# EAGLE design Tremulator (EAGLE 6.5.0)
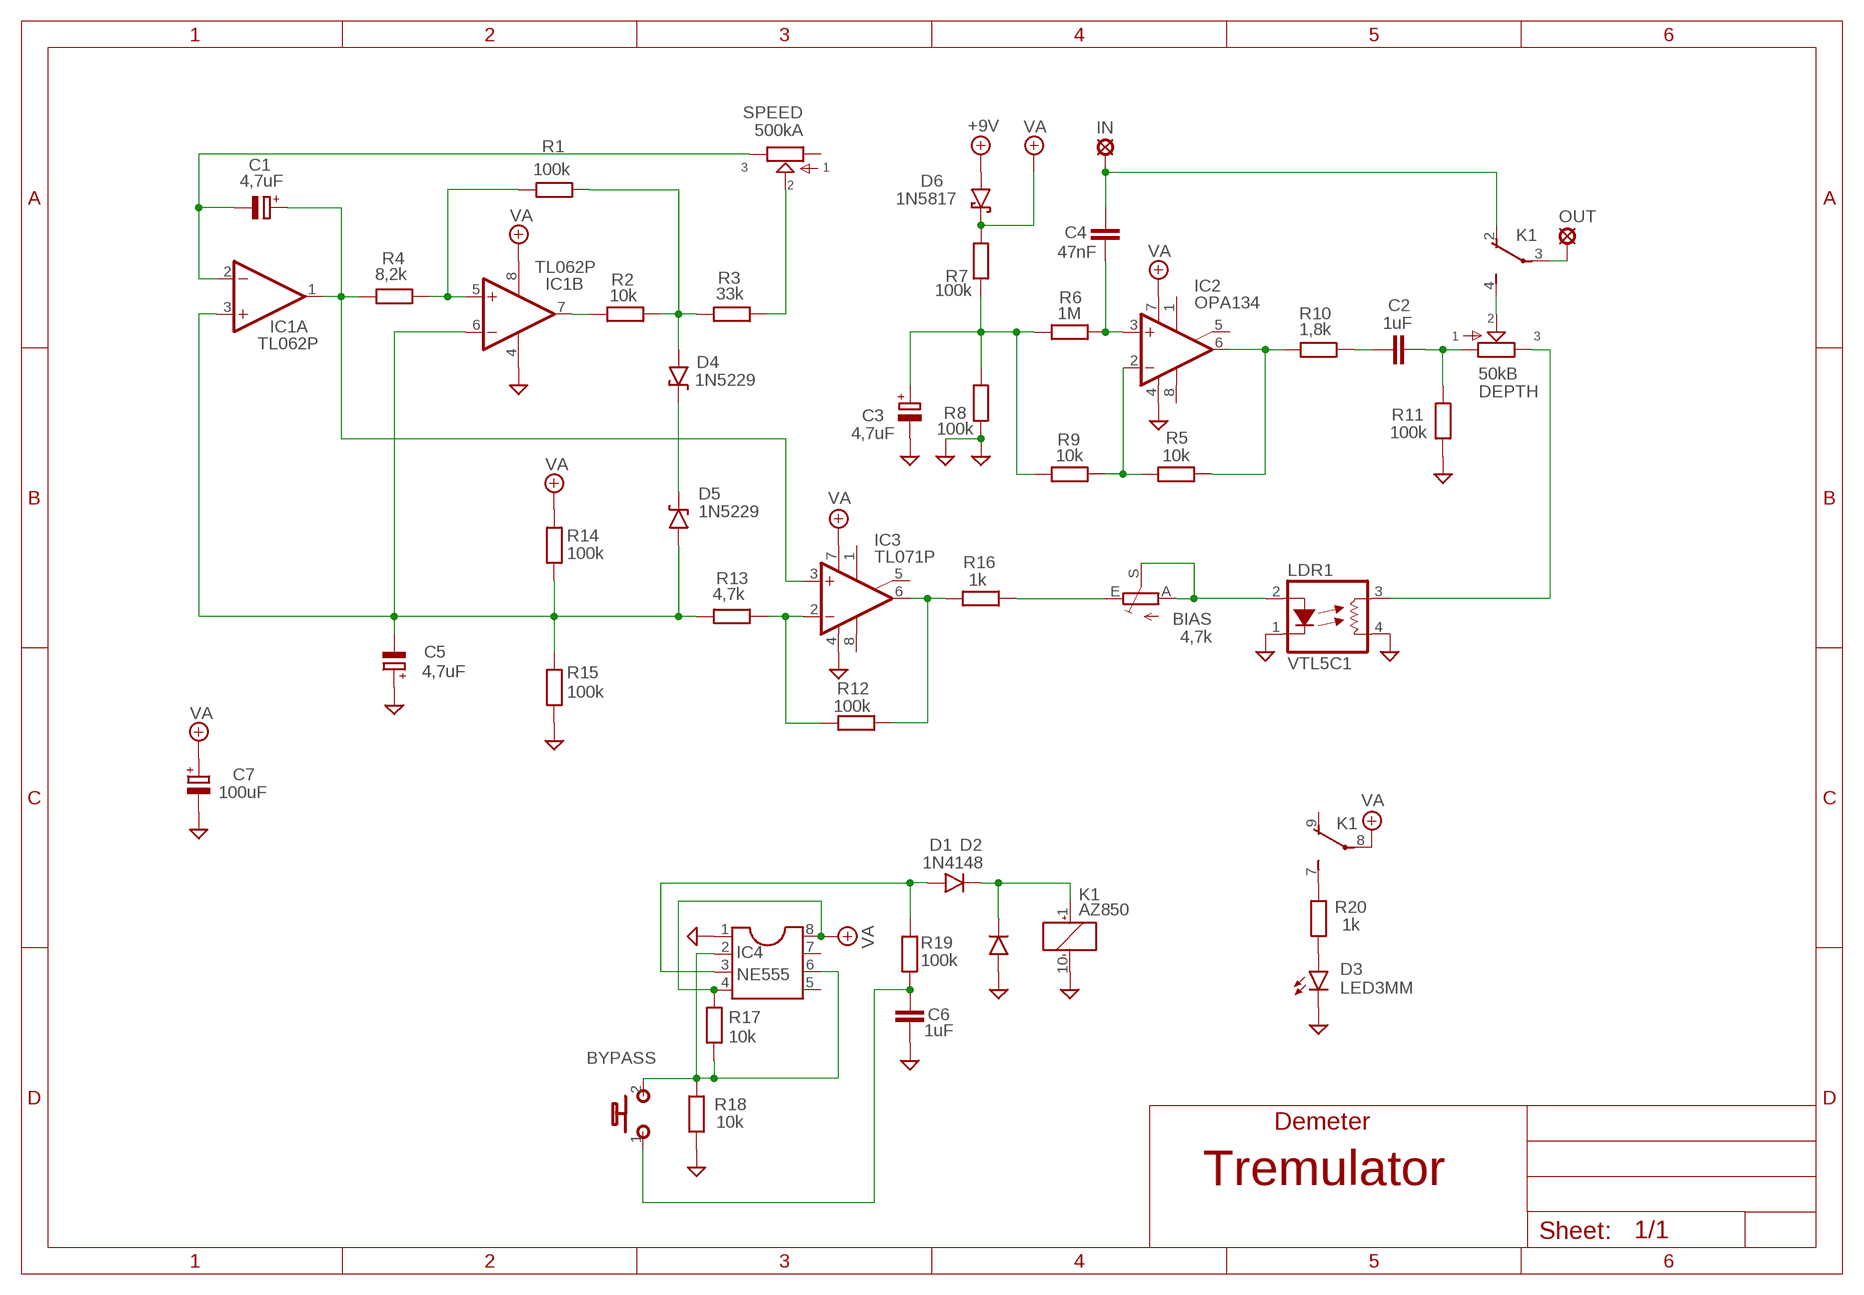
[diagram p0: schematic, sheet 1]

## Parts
+9V  +9V  +9V(T)1  [ROUND]
BIAS  4,7k  TRIM_EU-PT10  [PT-10]
BYPASS  MOMENTARY  [SPST]
C1  4,7uF  CPOL-EUB  [PANASONIC_B]
C2  1uF  072X0352  [072X035]
C3  4,7uF  CPOL-EUB  [PANASONIC_B]
C4  47nF  22NF-82NF"  [4,5MM]
C5  4,7uF  CPOL-EUB  [PANASONIC_B]
C6  1uF  072X0352  [072X035]
C7  100uF  CPOL-EUD  [PANASONIC_D]
D1  1N4148  1N4148-3  [DO35-3]
D2  1N4005  1N4148-3  [DO35-3]
D3  LED3MM  [LED3MM]
D4  1N5229  1N9ZENER  [DO35-3]
D5  1N5229  1N9ZENER  [DO35-3]
D6  1N5817  [DO41-3]
DEPTH  50kB  POT-EU16MM  [16MM]
GND  GND(T)1  [ROUND]
GND18  GND(T)1  [ROUND]
IC1  TL062P  [DIL08]
IC2  OPA134  TL071P  [DIL08]
IC3  TL071P  [DIL08]
IC4  NE555  DIL8  [DIL08]
IN  MCS10B  [MCS10B]
K1  AZ850  TQ2-5V  [TQ2]
LDR1  VTL5C1  VACTROL_4PIN  [VACTROL_4PIN_VTL5C]
OUT  MCS10B  [MCS10B]
R1  100k  6MM-EU3  [R0207/3]
R2  10k  6MM-EU3  [R0207/3]
R3  33k  6MM-EU3  [R0207/3]
R4  8,2k  6MM-EU3  [R0207/3]
R5  10k  6MM-EU3  [R0207/3]
R6  1M  6MM-EU3  [R0207/3]
R7  100k  6MM-EU3  [R0207/3]
R8  100k  6MM-EU3  [R0207/3]
R9  10k  6MM-EU3  [R0207/3]
R10  1,8k  6MM-EU3  [R0207/3]
R11  100k  6MM-EU3  [R0207/3]
R12  100k  6MM-EU3  [R0207/3]
R13  4,7k  6MM-EU3  [R0207/3]
R14  100k  6MM-EU3  [R0207/3]
R15  100k  6MM-EU3  [R0207/3]
R16  1k  6MM-EU3  [R0207/3]
R17  10k  6MM-EU3  [R0207/3]
R18  10k  6MM-EU3  [R0207/3]
R19  100k  6MM-EU3  [R0207/3]
R20  1k  6MM-EU3  [R0207/3]
SPEED  500kA  POT-EU16MM  [16MM]

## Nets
+9V: +9V.1(+9V) D6.A
GND: C3.- C5.+ C6.2 C7.- D2.A D3.K(C) GND18.1(GND) GND.1(GND) IC1.4(P:V-) IC2.4(V-) IC3.4(V-) IC4.1 K1.10(_:-) LDR1.1(LED-) LDR1.4(RES2) R8.1 R11.1 R15.1 R18.1
N$1: C1.- IC1.2(A:-IN) SPEED.3
N$2: C1.+ IC1.1(A:OUT) IC3.3(+IN) R4.1
N$3: IC1.5(B:+IN) R1.1 R4.2
N$4: IC1.7(B:OUT) R2.1
N$5: D4.A R1.2 R2.2 R3.1
N$6: R3.2 SPEED.2
N$7: IC2.2(-IN) R5.1 R9.2
N$8: IC2.6(OUT) R5.2 R10.1
N$9: C4.2 IC2.3(+IN) R6.2
N$10: C3.+ R6.1 R7.1 R8.2 R9.1
N$11: C2.1 R10.2
N$12: C2.2 DEPTH.1 R11.2
N$13: C4.1 IN.MP K1.2(1:O)
N$14: DEPTH.2 K1.4(1:S)
N$15: IC3.6(OUT) R12.2 R16.1
N$16: IC3.2(-IN) R12.1 R13.2
N$17: BIAS.E R16.2
N$18: DEPTH.3 LDR1.3(RES1)
N$19: D4.C D5.C
N$21: BIAS.A BIAS.S LDR1.2(LED+)
N$22: BYPASS.2(S) IC4.2 IC4.6 R17.1 R18.2
N$23: K1.3(1:P) OUT.MP
N$24: D1.A IC4.3 R19.2
N$25: BYPASS.1(P) C6.1 R19.1
N$26: D1.C D2.C K1.1(_:+)
N$27: K1.7(2:S) R20.2
N$28: D3.A R20.1
N$30: C5.- D5.A IC1.3(A:+IN) IC1.6(B:-IN) R13.1 R14.1 R15.2
VA: C7.+ D6.C IC1.8(P:V+) IC2.7(V+) IC3.7(V+) IC4.4 IC4.8 K1.8(2:P) R7.2 R14.2 R17.2
Unconnected: IC2.1(ON1) IC2.5(ON2) IC2.8(OPT) IC3.1(ON1) IC3.5(ON2) IC3.8(OPT) IC4.5 IC4.7 K1.9(2:O) SPEED.1

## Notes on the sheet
- Demeter

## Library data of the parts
+9V = Virransyöttö:+9V(T): +9V Voltage Supply
BIAS = pot:TRIM_EU-: POTENTIOMETER
BYPASS = Kytkimet:MOMENTARY
C1 C3 C5 C7 = rcl:CPOL-EU: POLARIZED CAPACITOR, European symbol
C2 C6 = Wima MKS:072X035: 0.15 - 1.0uF;
C4 = Mylar Kondensaattorit:22NF-82NF: 22nF-82nF
D1 D2 = Diodit:1N4148: Fast Switching Diode
D3 = Diodit:LED
D4 D5 = Diodit:1N9*ZENER: 1N9???B Zener Diode
D6 = Diodit:1N5817
DEPTH SPEED = potentiometers:POT-EU
GND GND18 = Virransyöttö:GND(T): Ground
IC1 = Operaatiovahvistimet:TL062: OP AMP
IC2 IC3 = Operaatiovahvistimet:TL071: OP AMP
IC4 = ic-package:DIL8: Dual In Line / Socket
IN OUT = Padit:MCS10B: SOLDER PAD
K1 = relay:TQ2?*: LOW PROFILE 2 FORM C RELAY NAiS Source: http://www.mew-europe.com/.. en_ds_61020_0001.pdf Source: http://www.mew-europe.com/.. en_ds_61020_0004.pdf; MF: AROMAT/ MATSUSHITA; MPN: TQ2-5V; OC_FARNELL: 1175716; OC_NEWARK: 64K3200
LDR1 = MusicThingModular:VACTROL_4PIN: 4 Pin Vactrol Resistive Photocoupler
R1-R20 = gm-resistors:6MM-EU: 6mm Resistors (European schematic symbol)

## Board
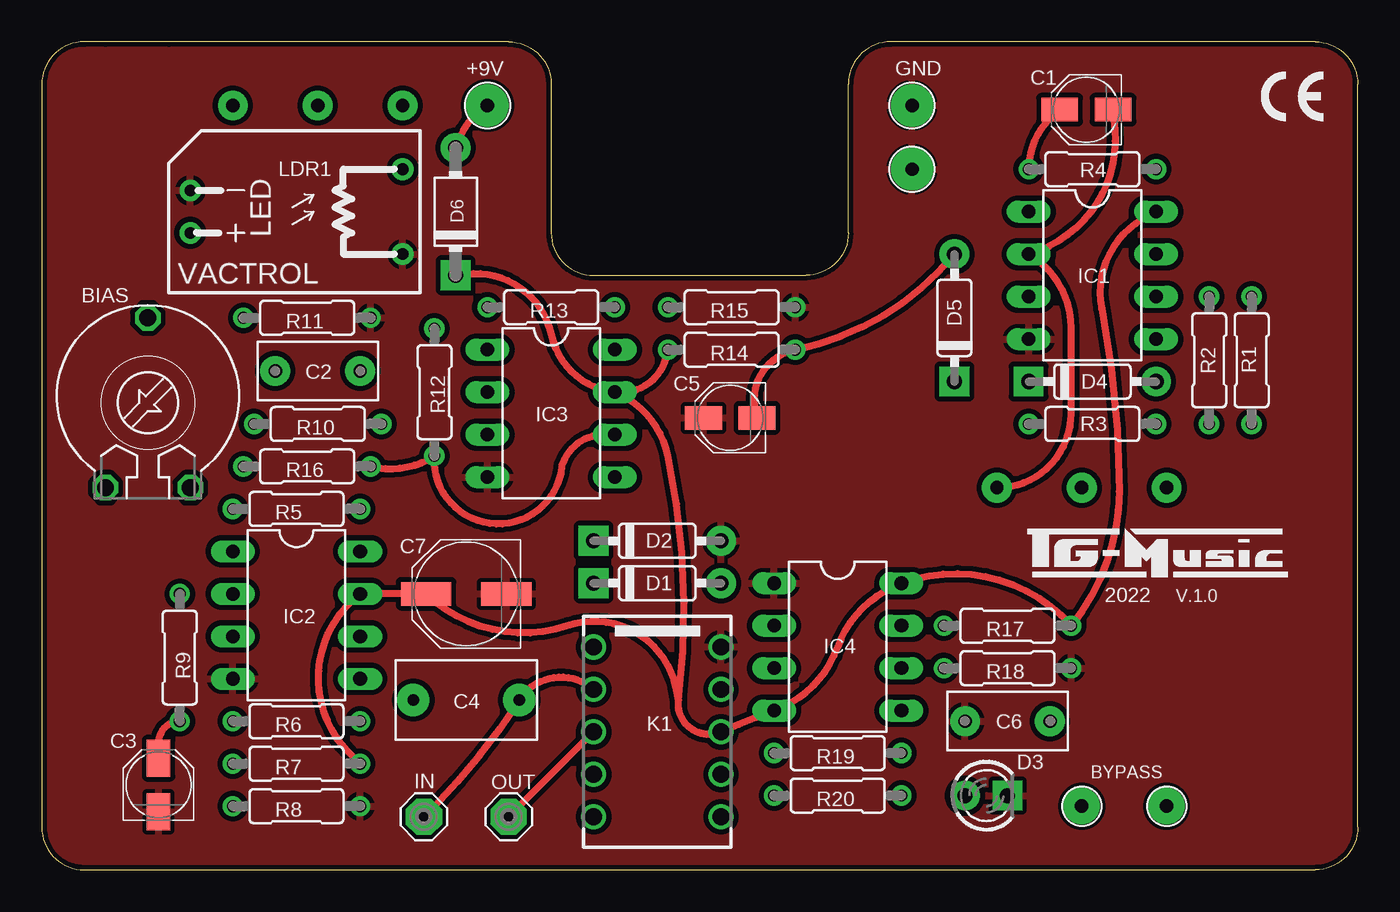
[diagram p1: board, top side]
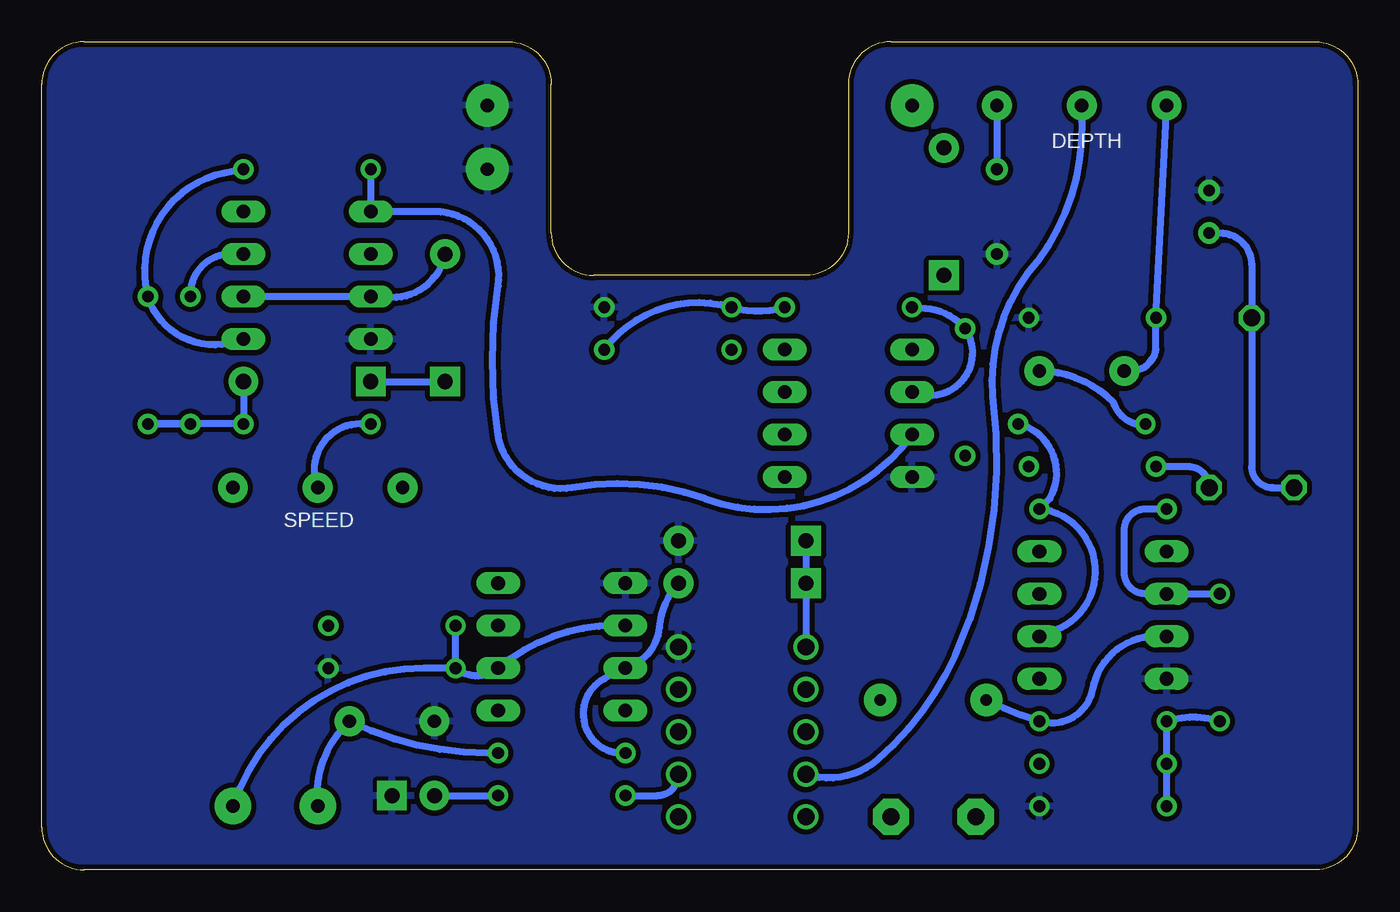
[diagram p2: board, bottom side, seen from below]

Size 78.74 x 49.53 mm. Coordinates in mm from the lower left corner, seen from the top.
Outline: 7.62,49.53 3.81,49.53
Outline: 78.74,2.54 78.74,46.99 arc90 76.2,49.53 50.8,49.53 arc90 48.26,46.99 48.26,38.1 arc-90 45.72,35.56 33.02,35.56 arc-90 30.48,38.1 30.48,46.99 arc90 27.94,49.53 2.54,49.53 arc90 0,46.99 0,2.54 arc90 2.54,0 76.2,0 arc90 78.74,2.54
Copper layers (1*16): Top 0.035mm / dielectric 1.5mm / Bottom 0.035mm
Design rules "ITEADstudio": minimum track width 10mil, minimum drill 12mil, track to track 12mil, track to pad 12mil, pad to pad 12mil, via to via 12mil, smd to smd 0mil, copper to edge 12mil, drill to drill 12mil, minimum pad ring 10mil, minimum via ring 6mil, stop-mask expansion 4mil, vias tented up to drill 100mil, thermal gap 10mil

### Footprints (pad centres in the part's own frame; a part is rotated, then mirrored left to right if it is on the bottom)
ROUND = drill 0.8 pad 2.54: 1 0,0
PT-10 = drill 1.016 octagon: A -2.54,-5.08; E 2.54,-5.08; S 0,5.08
SPST = drill 0.8 pad 2.184: 1 -2.54,0; 2 2.54,0
PANASONIC_B = smd 2.2 x 1.4: + 1.6,0; - -1.6,0
072X035 = drill 0.8 pad 1.778: 1 -2.54,0; 2 2.54,0
4,5MM = drill 0.7 pad 1.93: 1 -3.175,0; 2 3.175,0
PANASONIC_D = smd 3 x 1.4: + 2.4,0; - -2.4,0
DO35-3 = drill 0.9 pad 1.778: A 3.81,0 | drill 0.9 pad 1.778 square: C -3.81,0
LED3MM = drill 0.9 pad 1.778: A -1.27,0 | drill 0.9 pad 1.778 square: K 1.27,0
DO41-3 = drill 0.9 pad 1.778: A 3.81,0 | drill 0.9 pad 1.778 square: C -3.81,0
16MM = drill 0.8 pad 1.778: 1 5.08,0; 2 0,0; 3 -5.08,0
DIL08 = drill 0.813 long: 1 -3.81,-3.81; 2 -1.27,-3.81; 3 1.27,-3.81; 4 3.81,-3.81; 5 3.81,3.81; 6 1.27,3.81; 7 -1.27,3.81; 8 -3.81,3.81
MCS10B = drill 1.016 pad 2.159 octagon: MP 0,0
TQ2 = drill 1: 1 -5.08,-3.81; 2 -2.54,-3.81; 3 0,-3.81; 4 2.54,-3.81; 5 5.08,-3.81; 6 5.08,3.81; 7 2.54,3.81; 8 0,3.81; 9 -2.54,3.81; 10 -5.08,3.81
VACTROL_4PIN_VTL5C = drill 0.7 pad 1.3: 1 -6.35,1.27; 2 -6.35,-1.27; 3 6.35,2.54; 4 6.35,-2.54
R0207/3 = drill 0.7: 1 -3.81,0; 2 3.81,0

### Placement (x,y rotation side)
+9V  26.67,45.72 0 top
BIAS  6.35,27.94 0 top
BYPASS  64.77,3.81 0 top
C1  62.5,45.47 180 top
C2  16.51,29.84 180 top
C3  6.99,5.08 90 top
C4  25.4,10.16 180 top
C5  41.19,27.04 180 top
C6  57.78,8.89 180 top
C7  25.4,16.51 180 top
D1  36.83,17.14 0 top
D2  36.83,19.68 0 top
D3  56.52,4.45 0 top
D4  62.87,29.21 0 top
D5  54.61,33.02 90 top
D6  24.77,39.37 90 top
DEPTH  16.51,45.72 0 bottom
GND  52.07,45.72 0 top
GND18  52.07,41.91 0 top
IC1  62.87,35.56 270 top
IC2  15.24,15.24 270 top
IC3  30.48,27.3 270 top
IC4  47.62,13.34 270 top
IN  22.86,3.17 0 top
K1  36.83,8.26 270 top
LDR1  15.24,39.37 0 top
OUT  27.94,3.17 0 top
R1  72.39,30.48 270 top
R2  69.85,30.48 270 top
R3  62.87,26.67 180 top
R4  62.87,41.91 0 top
R5  15.24,21.59 0 top
R6  15.24,8.89 0 top
R7  15.24,6.35 0 top
R8  15.24,3.81 180 top
R9  8.26,12.7 90 top
R10  16.51,26.67 180 top
R11  15.88,33.02 180 top
R12  23.5,28.57 270 top
R13  30.48,33.66 180 top
R14  41.27,31.11 180 top
R15  41.27,33.66 180 top
R16  15.88,24.13 180 top
R17  57.78,14.61 0 top
R18  57.78,12.06 180 top
R19  47.62,6.99 180 top
R20  47.62,4.45 180 top
SPEED  62.23,22.86 180 bottom

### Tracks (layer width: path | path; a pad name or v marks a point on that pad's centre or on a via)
+9V
  Top 0.406: +9V.1 25.94,45.21 arc26 D6.A
GND
  pour Bottom: 0,2.54 0,46.99 arc-90 2.54,49.53 27.94,49.53 arc-90 30.48,46.99 30.48,38.1 arc90 33.02,35.56 45.72,35.56 arc90 48.26,38.1 48.26,46.99 arc-90 50.8,49.53 76.2,49.53 arc-90 78.74,46.99 78.74,2.54 arc-90 76.2,0 2.54,0 arc-90
  pour Top: 0,2.54 0,46.99 arc-90 2.54,49.53 27.94,49.53 arc-90 30.48,46.99 30.48,38.1 arc90 33.02,35.56 45.72,35.56 arc90 48.26,38.1 48.26,46.99 arc-90 50.8,49.53 76.2,49.53 arc-90 78.74,46.99 78.74,2.54 arc-90 76.2,0 2.54,0 arc-90
N$1
  Top 0.406: SPEED.3 arc90 61.59,27.3 61.59,32.38 arc59 IC1.2 arc79 64.2,44.24 C1.-
N$2
  Top 0.406: R4.1 59.12,42.46 arc-47 C1.+
  Bottom 0.406: R4.1 IC1.1 arc0 55.24,39.37 arc99 51.44,34.92 arc-18 51.44,26.04 arc-91 46.99,22.86 arc30 39.02,22.19 arc-74 IC3.3
N$3
  Bottom 0.406: R4.2 67.81,41.68 arc-93 R1.1 arc-90 67.16,31.6 IC1.5
N$4
  Bottom 0.406: IC1.7 67.42,36.83 arc-93 R2.1
N$5
  Bottom 0.406: D4.A R3.1 R1.2 R2.2
N$6
  Bottom 0.406: R3.2 59.69,26.67 arc-113 SPEED.2
N$7
  Bottom 0.406: R9.2 IC2.2 12.7,16.51 arc90 13.97,17.78 13.97,20.32 arc90 12.7,21.59 R5.1
N$8
  Bottom 0.406: R10.1 arc106 18.41,22.23 R5.2 arc153 18.12,14.33 IC2.6
N$9
  Bottom 0.406: IC2.3 12.06,13.97 arc-80 15.88,10.79 arc97 R6.2 arc8 C4.2
N$10
  Top 0.406: R9.1 arc90 6.99,7.62 C3.+
  Bottom 0.406: R8.2 R7.1 R6.1 arc34 R9.1
N$11
  Bottom 0.406: R10.2 13.34,26.67 arc53 14.61,27.94 arc-44 C2.1
N$12
  Bottom 0.406: C2.2 arc-90 12.06,31.11 R11.2 DEPTH.1
N$13
  Top 0.406: IN.MP 23.5,3.81 arc13 C4.1 arc-99 K1.2
N$14
  Bottom 0.406: DEPTH.2 16.52,44.76 arc39 19.18,36.38 arc-46 21.86,28.32 arc31 24.08,12.86 arc25 28.74,6.59 arc59 K1.4
N$15
  Top 0.406: R16.1 arc46 R12.2 arc178 31.11,24.13 arc-74 33.66,26.04 IC3.6
N$16
  Bottom 0.406: R13.2 25.85,33.59 arc45 R12.1 arc138 26.17,28.46 IC3.2
N$17
  Bottom 0.406: R16.2 10.16,24.13 arc90 BIAS.E
N$18
  Bottom 0.406: DEPTH.3 LDR1.3
N$19
  Bottom 0.406: D4.C D5.C
N$21
  Bottom 0.406: LDR1.2 8.26,38.1 arc90 6.35,36.2 BIAS.S 6.35,24.13 arc-90 5.08,22.86 BIAS.A
N$22
  Bottom 0.406: R18.2 55.88,12.06 arc-72 BYPASS.2 | IC4.2 44.45,14.61 arc-40 IC4.6 arc80 R18.2 | R18.2 R17.1
N$23
  Top 0.406: OUT.MP K1.3
N$24
  Bottom 0.406: D1.A arc-37 41.77,14.51 arc60 43.3,12.31 IC4.3 arc-2 45.09,11.43 arc-156 R19.2
N$25
  Bottom 0.406: BYPASS.1 arc53 C6.1 arc-26 52.07,6.99 R19.1
N$26
  Bottom 0.406: D2.C D1.C K1.1
N$27
  Bottom 0.406: R20.2 41.91,4.45 arc-90 K1.7
N$28
  Bottom 0.406: D3.A R20.1
N$30
  Top 0.406: C5.- 42.69,27.61 arc-88 R14.1 arc39 D5.A
  Bottom 0.406: D5.A arc90 58.42,34.29 IC1.3 IC1.6 | R14.1 arc69 R15.2 arc-33 R13.1
VA
  Top 0.406: R7.2 18.41,6.99 arc-98 IC2.7 C7.+ arc62 31.47,14.6 arc-96 37.94,10.91 38.1,10.16 | D6.C 25.39,35.64 arc-85 30.47,32.03 arc71 IC3.7 | IC3.7 arc90 R14.2 | 38.1,10.16 arc120 K1.8 arc-3 IC4.4 arc49 47.62,13.34 arc-49 IC4.8 arc-69 R17.2 arc39 64.46,22.64 arc11 63.42,33.55 arc-71 65.85,38.9 IC1.8 | 38.1,10.16 arc19 37.47,24.77 arc56 IC3.7

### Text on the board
tNames: 2022 | V.1.0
